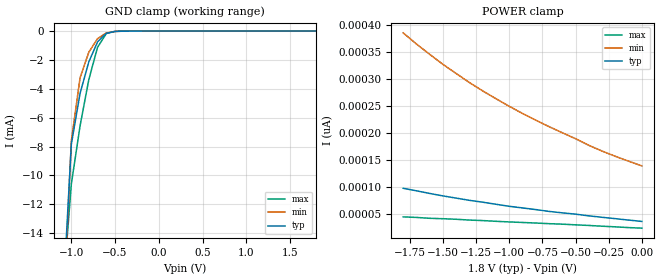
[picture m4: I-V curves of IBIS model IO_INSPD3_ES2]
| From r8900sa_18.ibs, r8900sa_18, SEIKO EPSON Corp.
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[Model]   IO_INSPD3_ES2
Model_type Input
Enable Active-Low
Polarity Non-Inverting
Vinh=1.44
Vinl=0.36
C_comp   2.5p   2p   3p
[Temperature Range] 25   85   -40
[Voltage Range]   1.8   1.6   2.0
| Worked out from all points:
|   GND clamp passes 1 mA (typ) near -0.72 V on its own axis
[GND Clamp]
-1.8V     -154.6mA   -131.5mA   -191.9mA
-1.1V     -19.18mA   -20.8mA    -18.39mA
-1V       -7.853mA   -7.611mA   -10.6mA
-900mV    -4.308mA   -3.238mA   -6.564mA
-800mV    -2.131mA   -1.46mA    -3.357mA
-700mV    -747.4uA   -523.1uA   -1.119mA
-600mV    -155uA     -130.4uA   -169.7uA
-500mV    -23.23uA   -25.44uA   -15.75uA
-400mV    -3.177uA   -4.273uA   -1.427uA
1.8V      37.06pA    157.3pA    21.94pA
[POWER Clamp]
-1.8V     98.34pA    385.6pA    45.47pA
-1.7V     93.68pA    365pA      44.45pA
-1.5V     84.24pA    327.4pA    42.06pA
-1.3V     76.06pA    293.8pA    39.56pA
-1.2V     72.65pA    278.3pA    38.65pA
-1V       65.03pA    249.8pA    36.15pA
-800mV    58.95pA    224.2pA    34.11pA
-400mV    47.35pA    177.7pA    29.62pA
-200mV    42.18pA    157.5pA    27.06pA
0V        37.06pA    139.8pA    24.61pA
